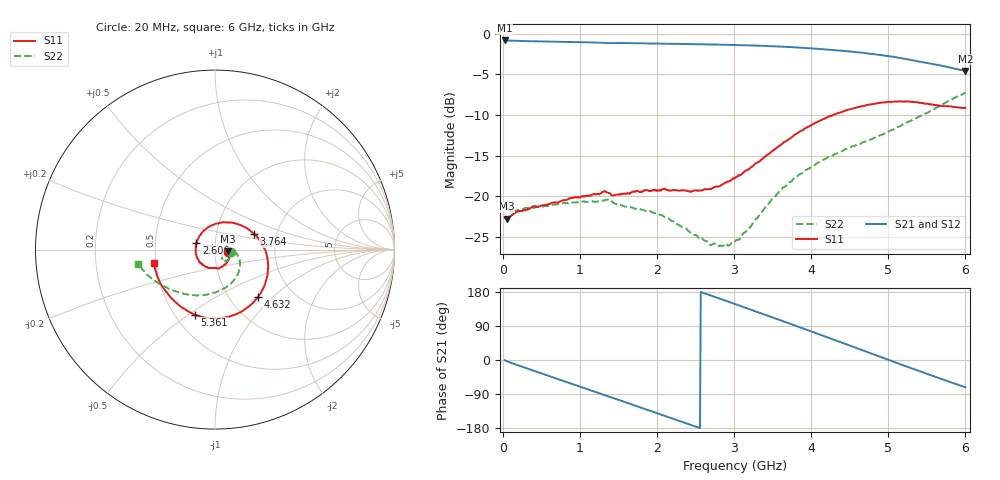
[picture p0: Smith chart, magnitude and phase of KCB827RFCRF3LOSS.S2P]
!Agilent Technologies,E5071B,JP1KK00126,A.08.11
!Date: Tue May 06 07:19:34 2014
!Data & Calibration Information:
!Freq	S11:SOLT2(ON)	S21:SOLT2(ON)	S12:SOLT2(ON)	S22:SOLT2(ON)
# Hz S dB R 50
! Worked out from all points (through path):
!   600 points, 20 MHz to 6 GHz, reference 50 ohm
!   highest |S21| = -0.83 dB at 20 MHz (marker M1); lowest = -4.6 dB at 6 GHz (marker M2)
!   group delay of S21, straight-line fit = 200 ps
!   lowest |S11| = -22.7 dB at 49.95 MHz (marker M3), VSWR 1.16, Z = 57.8 - j0.933 ohm
!   |S11| at or under -10 dB: start of sweep to 4.282 GHz
!   |S22| runs from -26.1 to -7.2 dB; largest |S21 - S12| = 0.0048
!   S11 on the Smith chart (normalised r, x): 20 MHz: 1.16, -0.04; 2.606 GHz: 0.81, +0.06; 3.764 GHz: 1.52, +0.28; 4.632 GHz: 1.35, -0.81; 5.361 GHz: 0.63, -0.53; 6 GHz: 0.49, -0.08
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2e7  -22.58 -12.4  -0.83 -0.7  -0.82 -0.8  -21.09 -9.6
4.994992e7  -22.74 -6.3  -0.83 -3.4  -0.83 -3.5  -21.37 -4.6
4.991987e8  -21.13 -23.4  -0.94 -35.4  -0.94 -35.4  -21.25 -11.7
7.687479e8  -20.53 -40.2  -1.01 -54.4  -1.01 -54.4  -20.86 -20.4
1.018331e9  -20.00 -56.1  -1.04 -71.7  -1.05 -71.8  -20.62 -27.9
1.247947e9  -19.74 -72.5  -1.09 -87.9  -1.09 -87.9  -20.60 -34.5
1.517496e9  -19.73 -92.6  -1.13 -106.6  -1.13 -106.6  -21.08 -44.2
1.757095e9  -19.37 -111.7  -1.17 -123.5  -1.16 -123.4  -21.47 -48.1
2.016661e9  -19.29 -134.6  -1.22 -141.7  -1.21 -141.7  -22.22 -52.1
2.31616e9  -19.29 -165.0  -1.26 -162.9  -1.26 -162.9  -23.71 -51.7
2.605676e9  -19.15 159.8  -1.31 176.7  -1.31 176.7  -25.39 -42.7
2.815326e9  -18.72 132.7  -1.34 161.8  -1.34 161.5  -26.03 -32.2
3.014992e9  -17.70 106.2  -1.39 147.3  -1.39 147.3  -25.49 -18.1
3.404341e9  -15.07 58.5  -1.50 119.1  -1.50 118.9  -21.29 -3.7
3.76374e9  -12.61 22.1  -1.66 92.8  -1.67 92.7  -17.88 -12.8
4.013322e9  -11.16 0.6  -1.80 74.4  -1.81 74.3  -16.27 -25.0
4.342771e9  -9.77 -25.6  -2.05 49.9  -2.05 49.7  -14.65 -46.1
4.632287e9  -8.97 -47.9  -2.32 28.2  -2.32 28.1  -13.53 -67.4
5.011653e9  -8.37 -77.1  -2.76 -0.3  -2.76 -0.4  -11.99 -98.3
5.361068e9  -8.42 -106.9  -3.35 -26.4  -3.35 -26.4  -10.39 -126.1
5.690518e9  -8.88 -137.1  -3.94 -50.2  -3.92 -50.2  -8.73 -148.9
6e9  -9.11 -168.0  -4.57 -72.1  -4.57 -72.0  -7.25 -169.1
